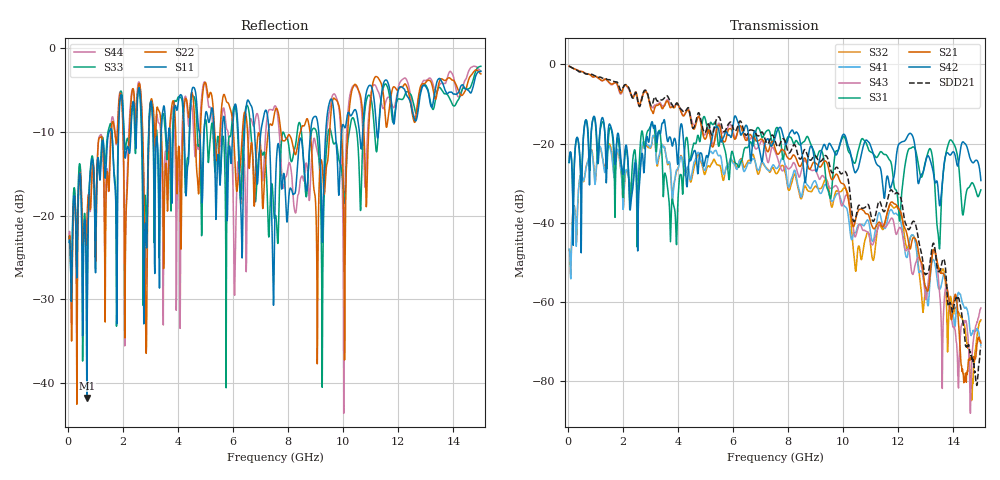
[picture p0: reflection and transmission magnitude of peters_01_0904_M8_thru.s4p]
# MHZ S RI R 50.00
! FREQ  S11  S12  S13  S14
!  S21  S22  S23  S24
!  S31  S32  S33  S34
!  S41  S42  S43  S44
!  REAL  IMAG  REAL  IMAG  REAL  IMAG  REAL  IMAG
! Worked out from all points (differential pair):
!   1496 points, 50 MHz to 15 GHz, reference 50 ohm
!   strongest paths, dB at 50 MHz, 3.79 GHz, 7.53 GHz, 11.27 GHz, 15 GHz:
!     S42: -24.7, -20.5, -18.4, -25.6, -29.3
!     S21: -0.4, -10.6, -21.3, -40.0, -70.3
!     S31: -24.8, -34.0, -16.9, -23.1, -31.7
!     S43: -0.4, -10.2, -22.1, -41.3, -61.5
!     S41: -46.6, -34.1, -26.0, -37.8, -70.9
!     S32: -46.8, -33.8, -27.2, -40.8, -64.5
!   taken as a pair (ports 1,3 in; 2,4 out), SDD21 dB: -0.4, -10.2, -19.4, -35.0, -71.2
!   lowest |S11| = -41.7 dB at 700 MHz (marker M1), VSWR 1.02, Z = 50.6 + j0.589 ohm
!   |S11| at or under -10 dB: start of sweep to 1.503 GHz; 3.105 GHz to 3.394 GHz (288.9 MHz wide, 8.89 % of centre); 7.307 GHz to 8.819 GHz (1.511 GHz wide, 18.7 % of centre)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
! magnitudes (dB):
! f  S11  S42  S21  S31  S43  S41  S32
! 50 MHz  -23.2  -24.7  -0.4  -24.8  -0.4  -46.6  -46.8
! 700 MHz  -41.7  -15.0  -2.4  -14.6  -2.4  -25.0  -25.0
! 3.08 GHz  -7.9  -14.7  -12.1  -15.3  -10.9  -18.3  -18.4
! 3.92 GHz  -6.9  -19.5  -10.2  -40.5  -10.1  -27.6  -27.8
! 4.95 GHz  -10.3  -25.6  -18.6  -13.1  -17.8  -26.6  -27.5
! 7.8 GHz  -16.0  -17.5  -21.5  -23.5  -26.9  -23.6  -25.5
! 15 GHz  -2.8  -29.3  -70.3  -31.7  -61.5  -70.9  -64.5
